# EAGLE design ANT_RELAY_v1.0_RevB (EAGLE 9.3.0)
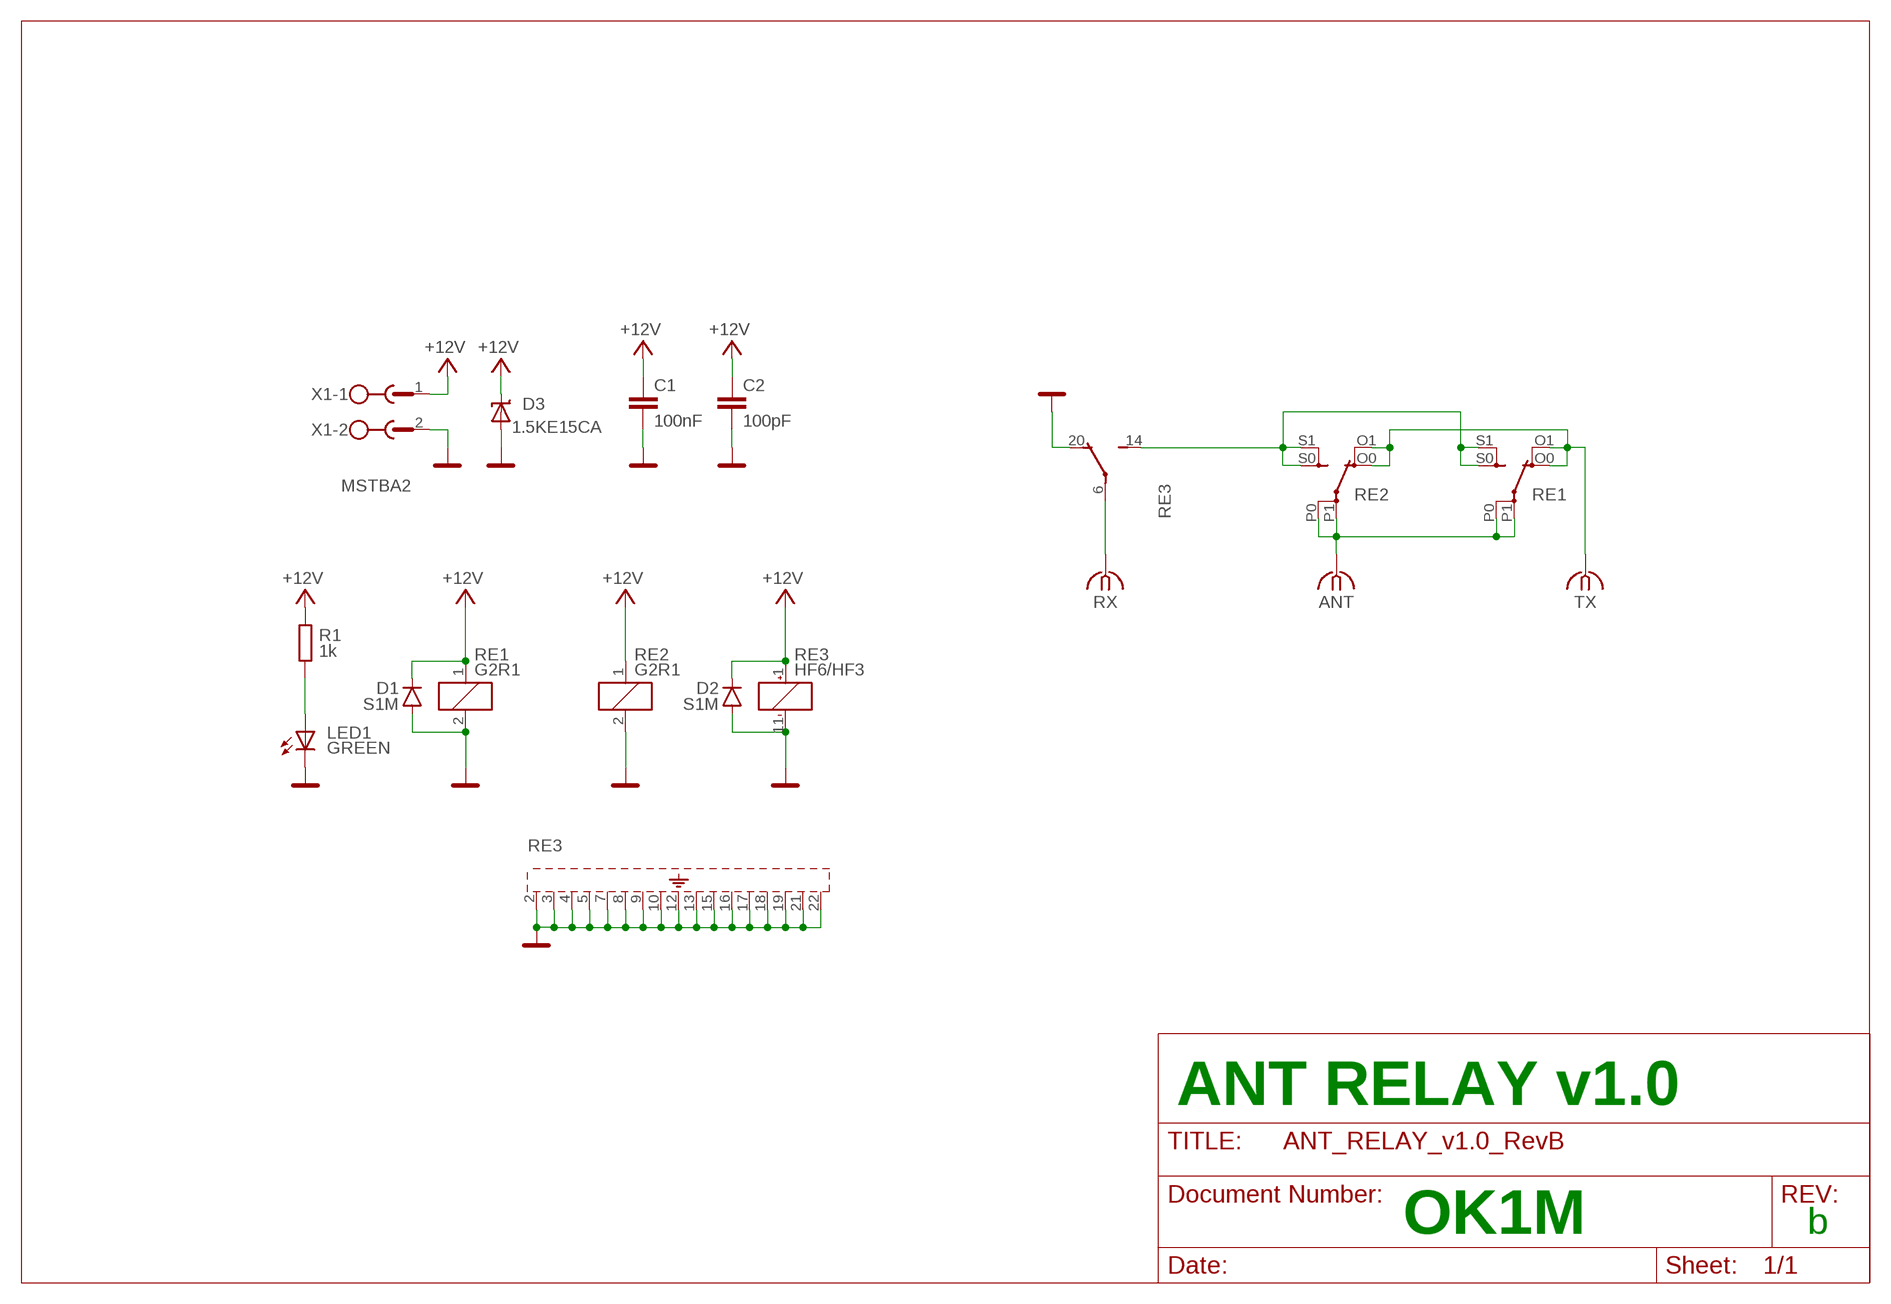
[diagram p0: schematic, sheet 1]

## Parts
ANT  N-180  [N-180]
C1  100nF  C-EUC0805  [C0805]
C2  100pF  C-EUC0805  [C0805]
D1  S1M  [SMA]
D2  S1M  [SMA]
D3  1.5KE15CA  TRANSILDO201-15  [DO201-15]
LED1  GREEN  LED3MM  [LED3MM]
R1  1k  R-EU_M0805  [M0805]
RE1  G2R1  G2RE  [G2RE]
RE2  G2R1  G2RE  [G2RE]
RE3  HF6/HF3  HF6-56+  [HF6-56]
RX  N-180  [N-180]
TX  N-180  [N-180]
X1  MSTBA2  [MSTBA2]

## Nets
+12V: C1.1 C2.1 D1.C D2.C D3.C R1.2 RE1.1 RE2.1 RE3.1 X1.1
ANT: ANT.1 RE1.P0(2:P) RE1.P1(2:P) RE2.P0(2:P) RE2.P1(2:P)
GND: C1.2 C2.2 D1.A D2.A D3.A LED1.K(C) RE1.2 RE2.2 RE3.2 RE3.3 RE3.4 RE3.5 RE3.7 RE3.8 RE3.9 RE3.10 RE3.11 RE3.12 RE3.13 RE3.15 RE3.16 RE3.17 RE3.18 RE3.19 RE3.20 RE3.21 RE3.22 X1.2
N$20: LED1.A R1.1
RX: RE3.6 RX.1
RX-ANT: RE1.S0(2:S) RE1.S1(2:S) RE2.S0(2:S) RE2.S1(2:S) RE3.14
TX: RE1.O0(2:O) RE1.O1(2:O) RE2.O0(2:O) RE2.O1(2:O) TX.1

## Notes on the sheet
- ANT RELAY v1.0
- OK1M | b

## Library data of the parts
ANT RX TX = #my:N-180
C1 C2 = rcl:C-EU: CAPACITOR, European symbol; SPICEPREFIX: C
D1 D2 = diode:S1M
D3 = #Marek:TRANSIL: TRANSIL
LED1 = led:LED: LED
R1 = rcl:R-EU_: RESISTOR, European symbol
RE1 RE2 = relay:G2RE: RELAY 1 x switch, high current, Omron; OC_FARNELL: unknown; OC_NEWARK: unknown
RE3 = #hf6-56:HF6-56+
X1 = con-phoenix-508:MSTBA2: PHOENIX; MF: FARNELL; MPN: 1757242; OC_FARNELL: 3705171; OC_NEWARK: 71C4161

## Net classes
0 default: width 0.203 mm, drill 0.406 mm, clearance 0.203 mm

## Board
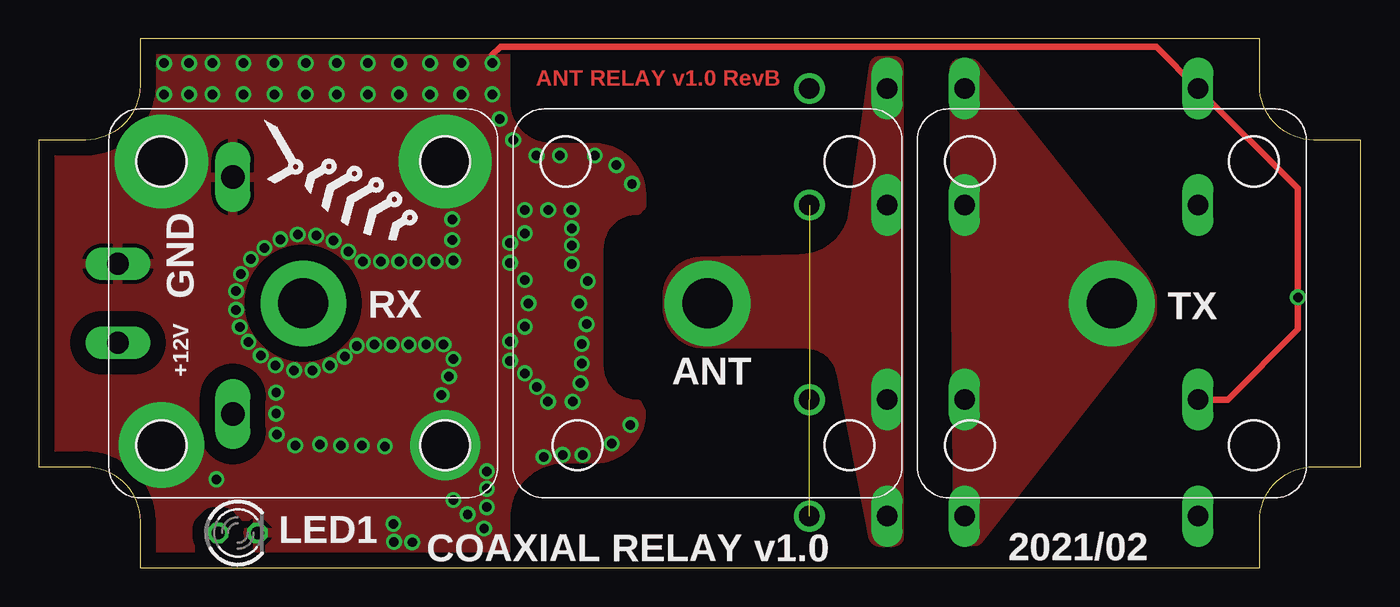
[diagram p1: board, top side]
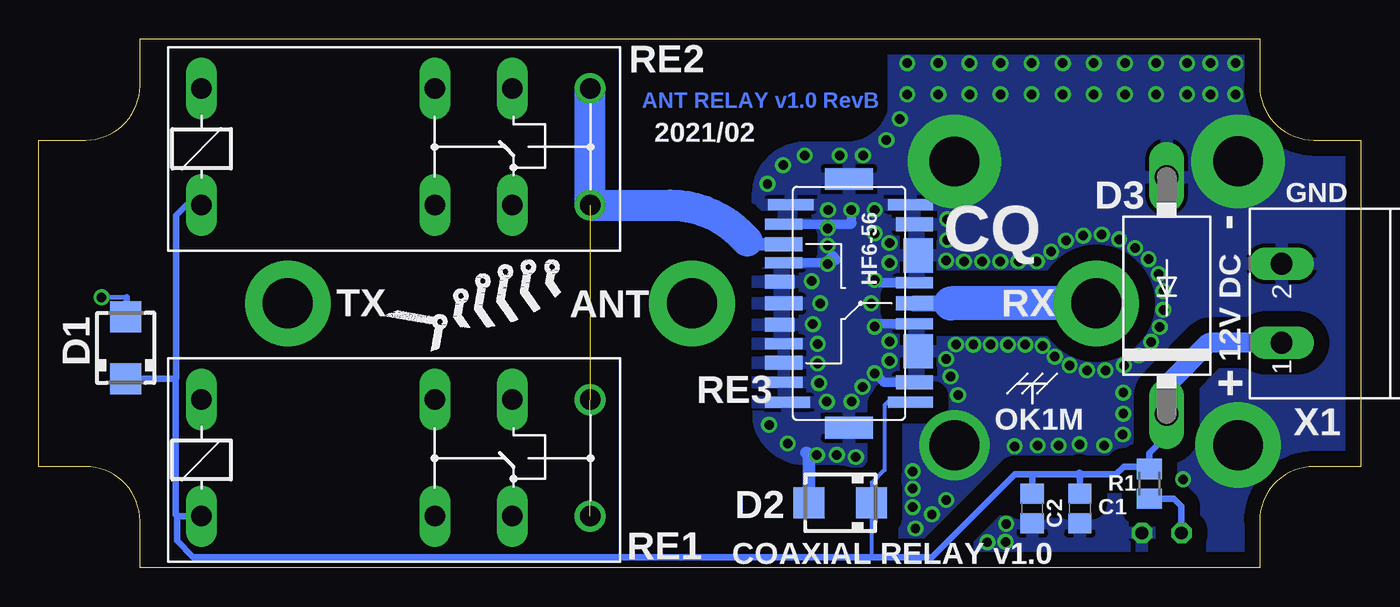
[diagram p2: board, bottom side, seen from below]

Size 85 x 34 mm. Coordinates in mm from the lower left corner, seen from the top.
Outline: 0,27.5 0,6.5 3,6.5 arc-90 6.5,3 6.5,0 78.5,0 78.5,3 arc-90 82,6.5 85,6.5 85,27.5 82,27.5 arc-90 78.5,31 78.5,34 6.5,34 6.5,31 arc-90 3,27.5 0,27.5
Copper layers (1*16): Top 0.035mm / dielectric 1.5mm / Bottom 0.035mm
Design rules "default *": minimum track width 10mil, minimum drill 24mil, track to track 8mil, track to pad 8mil, pad to pad 8mil, via to via 8mil, smd to smd 8mil, copper to edge 10mil, drill to drill 8mil, minimum pad ring 10mil, minimum via ring 8mil, stop-mask expansion 4mil, vias tented up to drill 0.7mm, thermal gap 10mil

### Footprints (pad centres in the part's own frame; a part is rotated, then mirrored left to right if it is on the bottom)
N-180 = drill 3.2 pad 5.5: 1 0,0
C0805 = smd 1.3 x 1.5: 1 -0.95,0; 2 0.95,0
SMA = smd 2 x 2: A 2,0; C -2,0
DO201-15 = drill 1.499 long: A 7.62,0; C -7.62,0
LED3MM = drill 0.813 octagon: A -1.27,0; K 1.27,0
M0805 = smd 1.3 x 1.6: 1 -0.95,0; 2 0.95,0
G2RE = drill 1.321 long: 1 -2.54,-3.683; 2 -2.54,3.81; O0 12.471,-3.683; O1 12.471,3.81; P0 17.45,-3.683; P1 17.45,3.81 | drill 1.321: S0 22.454,-3.683; S1 22.454,3.81
HF6-56 = smd 0.7 x 2.9: 1 -6.35,-3.95; 11 6.35,-3.95; 12 6.35,3.75; 22 -6.35,3.95 | smd 0.9 x 2.4: 2 -5.08,-4.2; 6 0,-4.2; 10 5.08,-4.2; 14 3.81,4.2; 17 0,4.2; 20 -3.81,4.2 | smd 2.2 x 1.9: 3 -3.075,-4.45; 8 3.075,-4.45 | smd 1.4 x 3.1: 4 -8,0; 9 8,0 | smd 0.7 x 2.4: 5 -1.317,-4.2; 7 1.317,-4.2; 13 5.08,4.2; 15 2.6,4.2; 19 -2.6,4.2; 21 -5.08,4.2 | smd 0.9 x 1.9: 16 1.375,4.45; 18 -1.375,4.45
MSTBA2 = drill 1.397 long: 1 -2.54,5.08; 2 2.54,5.08

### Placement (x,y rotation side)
ANT  43,17 0 top
C1  18.06,3.81 270 bottom
C2  21.12,3.81 270 bottom
D1  79.41,14.14 90 bottom
D2  33.47,4.18 180 bottom
D3  12.47,17.5 90 bottom
LED1  12.8,2.24 0 top
R1  13.59,5.39 90 bottom
RE1  72,7 0 bottom
RE2  72,27 0 bottom
RE3  32.9,17 90 bottom
RX  17,17 0 top
TX  69,17 0 top
U$1  [RYBICKA_12MM]  19.92,23.7 315 top
U$2  [RYBICKA_12MM]  55.43,17.09 5 bottom
X1  0,17 90 bottom

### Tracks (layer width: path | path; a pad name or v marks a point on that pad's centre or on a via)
+12V
  Bottom 0.254: RE3.1 30.41,10.65 30.61,10.45 30.61,6.3 31.43,5.48 31.43,4.22 D2.C 31.47,0.73 31.51,0.68
  Bottom 0.406: RE2.1 75.51,23.32 76.17,22.67 76.17,12.18 76.2,12.14 | D1.C 76.2,12.14 | 76.2,12.14 76.2,3.41 76.12,3.33 | 21.27,6 18.1,6 15.75,6 15.24,6.51 13.75,6.51 R1.2 13.59,7.37 12.47,8.48 D3.C 12.5,9.91 | 21.27,6 22.25,6 27.57,0.68 31.51,0.68 75.08,0.68 76.12,1.72 76.12,3.33 | C1.1 18.06,5.96 | C2.1 21.12,5.84 21.27,6 | RE1.1 76.1,3.32 76.12,3.33
  Bottom 0.61: 18.06,5.96 18.1,6
  Bottom 1.27: D3.C 12.47,11.74 9.75,14.46 X1.1
ANT
  pour Top (no thermals): 54.03,32.25 52.71,22.78 arc-80 49.06,19.52 42.53,19.34 arc88 40.75,17.51 40.75,16.75 arc90 42.75,14.75 49.28,14.75 arc-79 51.93,12.57 54,2 55,2 55,32.25
GND  (via drill 0.61, 3.2 pad 4.5, 3.2 pad 5.5, 3.2 pad 6)
  Top 0.406: RE1.2 76.45,10.81 80.96,15.32 v80.96,17.38 80.96,24.39 RE2.2 71.85,33.5 29.69,33.5 29.16,32.97 v29.16,32.44
  Bottom 0.305: 79.37,17.38 v80.96,17.38
  Bottom 0.406: 79.37,17.38 D1.A
  Bottom 0.61: RE3.7 31.07,18.32 v31.25,18.5 | RE3.5 31.07,15.68 v31.25,15.5 | RE3.13 32.77,22.08 32.7,22.15 32.75,22.19 v32.75,23 | RE3.15 33.98,19.6 33.81,19.76 33.73,19.76 33.73,19.84 33.97,20.08 34.27,19.78 v34.27,19.52 | RE3.2 30.67,11.92 v31.25,12.5
  Bottom 0.813: D2.A 35.47,7.21 35.5,7.25 | 35.64,7.38 35.5,7.25 | 35.5,7.25 v34.97,7.25
  other vias: 11.42,5.69 7.88,26.13 26.12,26.12 26.12,7.88 7.88,7.88 24.9,14.35 19.9,20.32 18.95,21.03 17.84,21.35 16.65,21.43 15.54,21.11 14.51,20.56 13.63,19.84 13,18.89 12.68,17.78 12.68,16.59 12.92,15.48 13.47,14.52 14.27,13.65 15.26,9.91 22.24,7.8 20.78,7.86 19.43,7.86 18.08,7.93 16.49,7.86 27.57,3.44 28.81,3.9 38.15,24.68 37.15,25.89 38.05,9.19 36.84,7.99 32.46,7.12 28.63,2.52 24,1.64 26.65,4.36 22.8,2.82 34.75,17 35.31,18.42 34.27,21.82 34.25,23 35.23,15.66 34.91,14.4 34.91,13.13 32.74,10.68 35.75,26.5 33.5,26.5 32,26.5 30.5,27.5 31.25,23 31.25,21.5 30.3,20.87 31.49,17 30.3,14.56 30.3,13.3 32.04,11.63 29.16,30.44 27.16,32.44 27.16,30.44 25.16,32.44 25.16,30.44 23.16,32.44 23.16,30.44 21.16,32.44 21.16,30.44 19.16,32.44 19.16,30.44 17.16,32.44 17.16,30.44 15.16,32.44 15.16,30.44 13.16,30.44 13.16,32.44 11.16,32.44 11.16,30.44 9.66,32.44 8.05,32.44 9.66,30.44 8.05,30.44 20.83,19.69 22,19.69 23.17,19.69 24.34,19.69 25.51,19.69 26.66,19.74 26.58,21.07 26.58,22.4 26.02,14.35 26.66,13.42 29.63,28.85 33.68,7.26 15.3,8.57 22.84,1.66 15.22,13.02 16.41,12.7 17.6,12.7 18.71,13.02 19.66,13.57 23.79,14.35 22.68,14.35 21.57,14.35 20.46,14.27 28.81,5.09 28.81,6.2 15.26,11.26 26.37,12.29 25.9,11.1 30.3,19.6 34.27,20.71 34.33,10.68 34.83,11.87
  pour Bottom (isolate 1): 0,0 30,0 30,3.25 arc-90 33.75,7 35.75,7 arc90 38.75,10 38.75,24 arc90 35.75,27 33,27 arc-90 30,30 30,34 0,34
  pour Top (isolate 1): 0,0 30,0 30,3.25 arc-90 33.75,7 35.75,7 arc90 38.75,10 38.5,10.5 arc-90 36,13 36,20.5 arc-90 38.5,23 38.75,23.25 38.75,24 arc90 35.75,27 33,27 arc-90 30,30 30,34 0,34
N$20
  Bottom 0.406: LED1.A 11.53,3.95 12.02,4.44 R1.1
RX
  Bottom 1.016: RE3.6 26.35,17 25.25,17 25.24,16.99
  Bottom 2.2: RX.1 26.35,17
RX-ANT  (2 unrouted)
  Bottom 0.406: 39.02,20.81 39.25,21.03
  Bottom 0.813: RE3.14 39,20.81 | 39,20.81 39.02,20.81 | 39.44,21 39.19,21 39,20.81
  Bottom 2: RE2.S1 RE2.S0 44.39,23.32 arc45 39.9,21.46 39.44,21
TX
  pour Top (no thermals): 71.3,16.75 arc-38 70.99,15.85 60.14,2 59.45,2 59.2,32.1 59.92,32.1 70.65,18.62 arc-39

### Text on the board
Top: ANT RELAY v1.0 RevB
Bottom: ANT RELAY v1.0 RevB
tPlace: GND | +12V | COAXIAL RELAY v1.0 | 2021/02
bPlace: 2021/02 | GND | - | CQ | 12V DC | RX | ANT | TX | + | OK1M | COAXIAL RELAY v1.0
